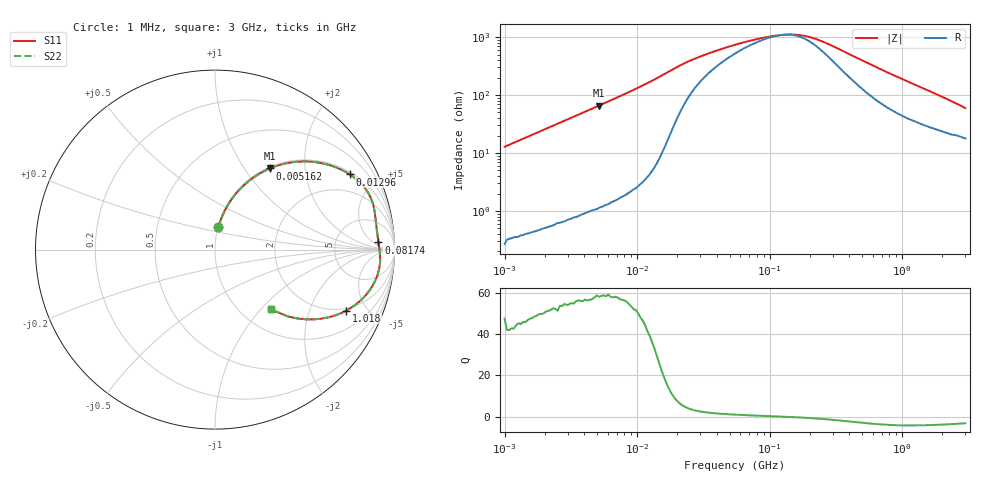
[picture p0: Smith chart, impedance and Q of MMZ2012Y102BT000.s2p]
! S-parameter Generated by TDK Corporation
! Copyright(C) 2016 TDK Corporation.
! All Rights Reserved.
! TDK P/N: MMZ2012Y102BT000 (Chip Beads)
! Property: |Z|=1000¶ at 100MHz
! Size(LxWxT): 2x1.25x0.85mm, 0.079x0.049x0.033inches
! Model Type: s2p (Touchstone File Format Version 1.0)
! Frequency: DC=Yes Start=1MHz Stop=3000MHz 202points Log-sweep
! Note: This model was converted from impedance.
! Model Generated on May. 16, 2016
! Hash(MD5):
! Port Assignments:
!  1 ---@@@--- 2
! Applicable Conditions:
!  Temperature = 25 degC
!  DC Bias Current = 0 A
!  Small Signal Operation
! Terms and conditions regarding TDK Simulation Models
! (1)This simulation model is being provided solely for informational purposes. Please refer to the specifications of the products in terms of detailed characteristics of such products.
! (2)In no event shall TDK Corporation of any of its subsidiaries be liable for any loss or damage arising, directly or indirectly,
!  From any information contained in this simulation model, including, but not limited to loss or damages arising from any inaccuracies, omissions or errors in connection with such information.
! (3)Any and all copyrights on this simulation model are owned by TDK Corporation.
!  Duplication or redistribution of this simulation model without prior written permission from TDK Corporation is prohibited.
! (4)This simulation model is subject to any modification or change without any prior notice.
! (5)Neither TDK Corporation nor any of its subsidiaries shall make any warranty, express or implied,
!  Including but not limited to the correctness, implied warranties of merchantability and fitness for a particular purpose with respect to this simulation models.
! (6)The use of this simulation model shall be deemed to have consented to the terms and conditions hereof.
# MHz S MA R 50
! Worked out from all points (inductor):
!   201 points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, 1 MHz to 3 GHz, reference 50 ohm
!   read as one part in series: L = 2.04 uH near 1.041 MHz
!   highest Q = 58.4 at 5.162 MHz (marker M1), where L = 2.03 uH
!   self-resonance near 128.6 MHz
!   S11 on the Smith chart (normalised r, x): 1 MHz: 1.01, +0.26; 5.162 MHz: 1.02, +1.32; 12.96 MHz: 1.10, +3.53; 81.74 MHz: 18, +8; 1.018 GHz: 1.86, -3.61; 3 GHz: 1.36, -1.13
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1  0.1268 81.5  0.9893 -7.3  0.9893 -7.3  0.1268 81.5
2.226959  0.2719 73.1  0.9571 -15.8  0.9571 -15.8  0.2719 73.1
3.900413  0.4414 62.8  0.8895 -26.2  0.8895 -26.2  0.4414 62.8
5.161903  0.5454 56.0  0.8288 -33.0  0.8288 -33.0  0.5454 56.0
6.563319  0.6383 49.4  0.7588 -39.7  0.7588 -39.7  0.6383 49.4
8.345207  0.7273 42.3  0.6733 -46.7  0.6733 -46.7  0.7273 42.3
12.9622  0.8598 29.2  0.4873 -59.3  0.4873 -59.3  0.8598 29.2
14.61624  0.8851 25.6  0.4329 -62.2  0.4329 -62.2  0.8851 25.6
19.34349  0.9148 18.1  0.3131 -65.4  0.3131 -65.4  0.9148 18.1
26.64524  0.9124 12.1  0.2199 -60.6  0.2199 -60.6  0.9124 12.1
54.77226  0.9089 5.0  0.1234 -40.0  0.1234 -40.0  0.9089 5.0
81.73662  0.9117 2.5  0.09779 -24.2  0.09779 -24.2  0.9117 2.5
108.1723  0.9145 1.0  0.087 -10.2  0.087 -10.2  0.9145 1.0
143.1579  0.9179 -0.6  0.08277 7.2  0.08277 7.2  0.9179 -0.6
174.8812  0.9201 -1.9  0.08604 20.8  0.08604 20.8  0.9201 -1.9
213.6344  0.9219 -3.3  0.0961 34.0  0.0961 34.0  0.9219 -3.3
457.0858  0.9081 -11.2  0.2081 58.3  0.2081 58.3  0.9081 -11.2
800.5644  0.8504 -20.3  0.3581 55.6  0.3581 55.6  0.8504 -20.3
1017.911  0.8058 -25.0  0.4343 51.6  0.4343 51.6  0.8058 -25.0
1782.824  0.6498 -36.7  0.6172 39.0  0.6172 39.0  0.6498 -36.7
2359.433  0.5487 -42.6  0.7026 31.9  0.7026 31.9  0.5487 -42.6
3000  0.4546 -46.8  0.7647 25.7  0.7647 25.7  0.4546 -46.8
